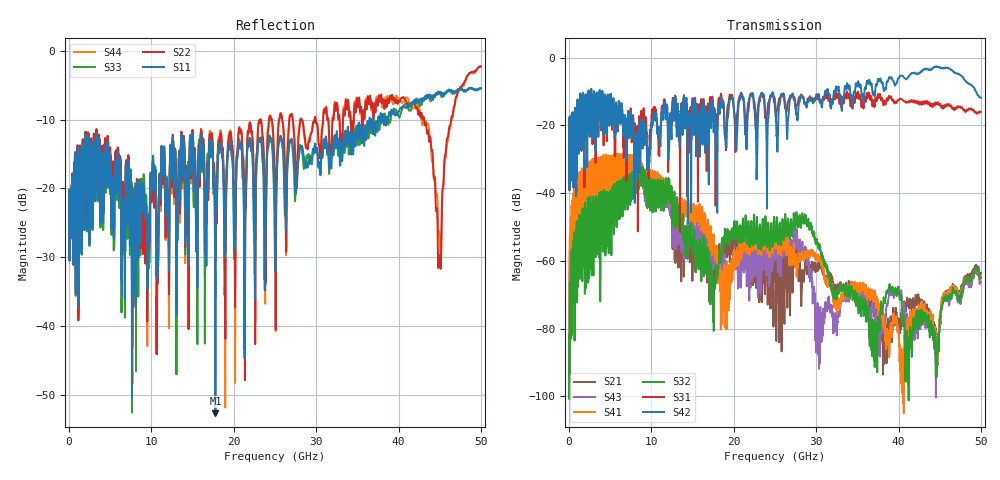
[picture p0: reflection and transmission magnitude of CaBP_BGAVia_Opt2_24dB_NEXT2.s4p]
!* Samtec Inc. NovaRay Examax Flyover System  *
!*  REV DATE  = 08/08/18  *
!*  TYPE  = TOUCHSTONE  *
!*  PORTS  = 4 port  *
!*  UNITS  = GHz  *
!*  DATA RANGE = DC  to 50 GHz; 10 MHz Step  *
!*  PARAMETER  = S  *
!*  FORMAT  = Real-Imaginary  *
!*  REFERENCE  = 50 ohms  *
!*  SOURCE  = HFSS  *
!*  VALIDATED  = No  *
!*  MANUFACTURER = SAMTEC  *
!*  INTERCONNECT = NVAx to EBCx to EBCx to NVAx  *
!*  [Full Channel NVAx to EBCx to EBCx to NVAx  with PCB Trace and BGA Via]  *
!*  BOUNDARY A  = Silicon BGA Ball Pad  *
!*  BOUNDARY B  = Silicon BGA Ball Pad  *
!*  NVAx (end a) ->>- (end b) NVAx  *
!*  Port 01 ->>- Port 02  *
!*  Port 03 ->>- Port 04  *
!***************************** CHANNEL MODEL ******************************************
# GHz S RI R 50
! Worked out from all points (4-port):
!   5000 points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, 10 MHz to 50 GHz, reference 50 ohm
!   strongest paths, dB at 10 MHz, 12.51 GHz, 25.01 GHz, 37.51 GHz, 50 GHz:
!     S42: -23.2, -15.3, -12.7, -6.2, -11.8
!     S31: -23.2, -14.5, -15.2, -10.7, -16.0
!     S32: -85.4, -42.3, -54.1, -81.6, -64.8
!     S41: -71.9, -46.9, -55.1, -71.7, -64.8
!     S43: -75.6, -50.2, -58.9, -85.6, -66.1
!     S21: -76.7, -51.1, -62.5, -74.9, -63.6
!   lowest |S11| = -52.7 dB at 17.77 GHz (marker M1), VSWR 1.00, Z = 49.8 - j0.145 ohm
!   |S11| at or under -10 dB: start of sweep to 36.46 GHz; 36.55 GHz to 36.75 GHz (204 MHz wide, 0.557 % of centre); 36.79 GHz to 37.51 GHz (722.9 MHz wide, 1.95 % of centre)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
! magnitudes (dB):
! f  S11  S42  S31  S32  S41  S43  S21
! 10 MHz  -22.7  -23.2  -23.2  -85.4  -71.9  -75.6  -76.7
! 1.66 GHz  -13.6  -10.4  -10.8  -49.1  -35.1  -39.5  -40.9
! 8.63 GHz  -26.2  -33.5  -33.9  -32.1  -30.1  -32.0  -32.0
! 17.77 GHz  -52.7  -19.7  -28.1  -65.4  -59.3  -61.6  -66.9
! 28.51 GHz  -15.5  -12.3  -12.6  -47.7  -59.5  -57.4  -64.4
! 44.98 GHz  -6.2  -3.0  -13.9  -80.7  -78.0  -78.8  -79.5
! 50 GHz  -5.5  -11.8  -16.0  -64.8  -64.8  -66.1  -63.6
